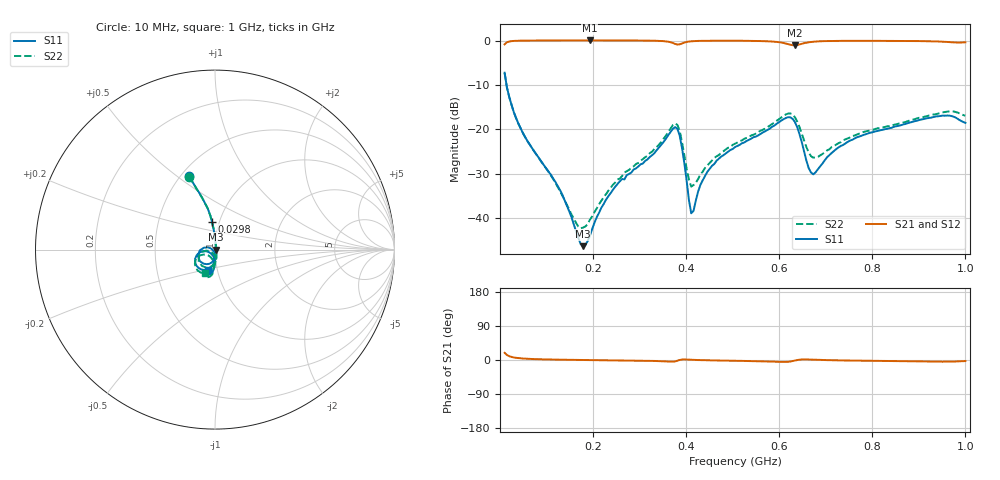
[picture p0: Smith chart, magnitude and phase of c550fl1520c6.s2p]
!Agilent Technologies,N5234A,MY52241123,A.10.00.00
!Agilent N5234A: A.10.00.00
!Date: Monday, August 26, 2019 10:03:40
!Correction: S11(Full 2 Port(1,2))
!S21(Full 2 Port(1,2))
!S12(Full 2 Port(1,2))
!S22(Full 2 Port(1,2))
!S2P File: Measurements: S11, S21, S12, S22:
# Hz S  dB  R 50
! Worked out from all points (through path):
!   201 points, 10 MHz to 1 GHz, reference 50 ohm
!   highest |S21| = 0.03 dB at 193.2 MHz (marker M1); lowest = -1.1 dB at 633.7 MHz (marker M2)
!   lowest |S11| = -46.3 dB at 178.3 MHz (marker M3), VSWR 1.01, Z = 50.5 + j0.0445 ohm
!   |S11| at or under -10 dB: 14.15 MHz to end of sweep
!   |S22| runs from -42.3 to -7.3 dB; largest |S21 - S12| = 0.002
!   S11 on the Smith chart (normalised r, x): 10 MHz: 0.55, +0.55; 29.8 MHz: 0.92, +0.29; 1 GHz: 0.90, -0.21
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1e7  -7.24 109.5  -0.85 18.9  -0.84 19.0  -7.29 109.6
2.98e7  -16.14 96.3  -0.08 6.7  -0.08 6.7  -16.12 96.4
1.288e8  -33.62 78.0  0.02 0.8  0.02 0.8  -33.84 73.0
1.684e8  -44.38 37.9  0.03 0.2  0.02 0.2  -41.87 23.4
1.783e8  -46.29 5.2  0.03 0.1  0.02 0.1  -42.12 -0.6
1.9315e8  -43.98 -41.1  0.03 -0.2  0.02 -0.1  -40.34 -31.5
2.179e8  -37.63 -67.2  0.02 -0.5  0.02 -0.5  -36.04 -56.7
2.476e8  -32.92 -78.2  0.02 -0.9  0.02 -0.9  -31.97 -70.1
3.4165e8  -24.09 -99.4  -0.06 -2.9  -0.07 -2.9  -23.43 -88.2
3.8125e8  -19.87 -159.9  -0.90 -2.0  -0.90 -2.0  -18.98 -143.7
3.9115e8  -24.19 169.9  -0.64 1.2  -0.65 1.2  -22.83 -169.8
4.1095e8  -38.89 -152.3  -0.16 0.7  -0.17 0.6  -32.88 -141.2
4.456e8  -29.53 -87.9  -0.04 -0.7  -0.05 -0.7  -28.11 -91.1
5.05e8  -23.98 -90.8  -0.04 -2.0  -0.04 -2.0  -23.23 -88.2
6.139e8  -17.45 -124.8  -0.65 -5.1  -0.67 -5.1  -16.65 -116.6
6.337e8  -18.33 -155.7  -1.06 -1.5  -1.07 -1.4  -17.25 -144.8
6.634e8  -28.74 -156.5  -0.38 1.4  -0.39 1.4  -25.19 -147.6
6.733e8  -30.12 -130.3  -0.26 0.9  -0.27 0.9  -26.36 -132.6
7.327e8  -23.70 -91.5  -0.06 -1.1  -0.07 -1.1  -22.86 -97.2
8.3665e8  -19.72 -92.9  -0.06 -2.7  -0.07 -2.7  -19.23 -94.8
9.505e8  -16.90 -102.9  -0.25 -4.5  -0.25 -4.4  -16.18 -101.7
1e9  -18.52 -108.9  -0.39 -2.8  -0.39 -2.8  -16.93 -111.8
